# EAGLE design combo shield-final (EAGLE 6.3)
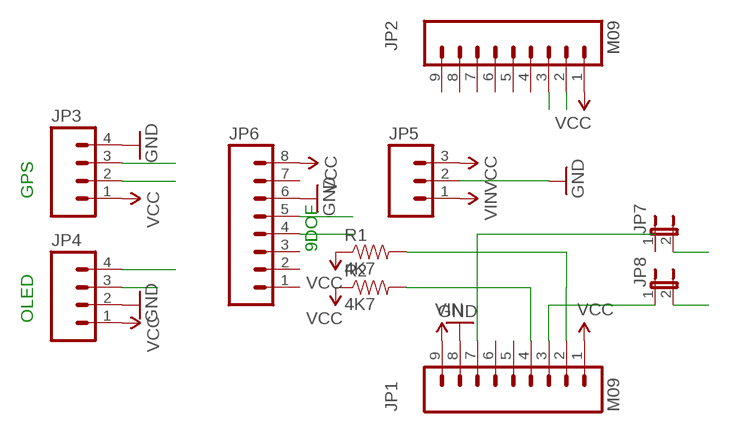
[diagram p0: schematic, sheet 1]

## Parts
JP1  M09  [1X09]
JP2  M09  [1X09]
JP3  M04PTH  [1X04]
JP4  M04PTH  [1X04]
JP5  M03PTH  [1X03]
JP6  M081X08  [1X08]
JP7  JUMPER-2SMD-NO  [SJ_2S-NO]
JP8  JUMPER-2SMD-NO  [SJ_2S-NO]
R1  4K7  RESISTORPTH-1/4W  [AXIAL-0.4]
R2  4K7  RESISTORPTH-1/4W  [AXIAL-0.4]

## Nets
GND [POWER]: JP1.8 JP3.4 JP4.2 JP5.2 JP6.6
N$2: JP1.3 JP8.1
N$3: JP1.7 JP7.1
RX: JP2.2 JP3.3 JP7.2
SCL: JP1.4 JP4.3 JP6.5 R2.P$2
SDA: JP1.2 JP4.4 JP6.4 R1.P$2
TX: JP2.3 JP3.2 JP8.2
VCC: JP1.1 JP2.1 JP3.1 JP4.1 JP5.3 JP6.8 R1.P$1 R2.P$1
VIN: JP1.9 JP5.1
Unconnected: JP1.5 JP1.6 JP2.4 JP2.5 JP2.6 JP2.7 JP2.8 JP2.9 JP6.1 JP6.2 JP6.3 JP6.7

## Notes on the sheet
- GPS
- 9DOF
- OLED

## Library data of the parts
JP1 JP2 = SparkFun:M09: Header 9 Standard 9-pin 0.1" header. Use with straight break away headers (SKU : PRT-00116), right angle break away headers (PRT-00553), swiss pins (PRT-00743), machine pins (PRT-00117), and female headers (PRT-00115).
JP3 JP4 = SparkFun-Connectors:M04: Header 4 Standard 4-pin 0.1" header. Use with straight break away headers (SKU : PRT-00116), right angle break away headers (PRT-00553), swiss pins (PRT-00743), machine pins (PRT-00117), and female headers (PRT-00115). Molex polarized connector foot print use with SKU : PRT-08231 with associated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
JP5 = SparkFun:M03: Header 3 Standard 3-pin 0.1" header. Use with straight break away headers (SKU : PRT-00116), right angle break away headers (PRT-00553), swiss pins (PRT-00743), machine pins (PRT-00117), and female headers (PRT-00115). Molex polarized connector foot print use with SKU : PRT-08232 with associated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
JP6 = SparkFun:M08: Header 8 Standard 8-pin 0.1" header. Use with straight break away headers (SKU : PRT-00116), right angle break away headers (PRT-00553), swiss pins (PRT-00743), machine pins (PRT-00117), and female headers (PRT-00115).
JP7 JP8 = SparkFun-Passives:JUMPER-2: Jumper
R1 R2 = SparkFun-Resistors:RESISTOR: Resistor

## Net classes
1 POWER: width 0.203 mm

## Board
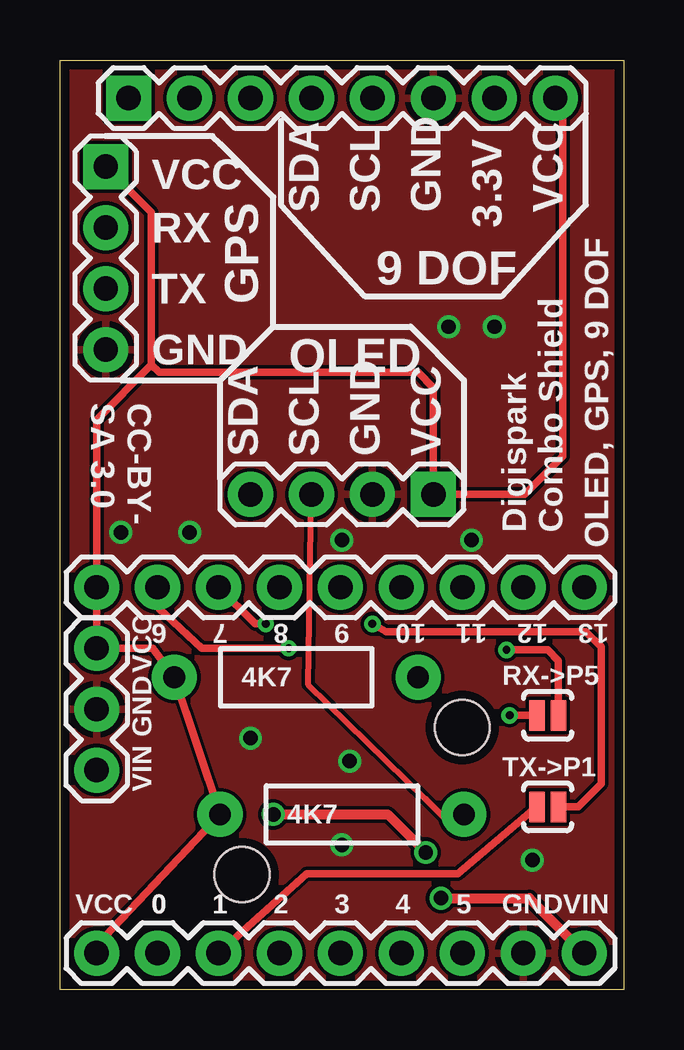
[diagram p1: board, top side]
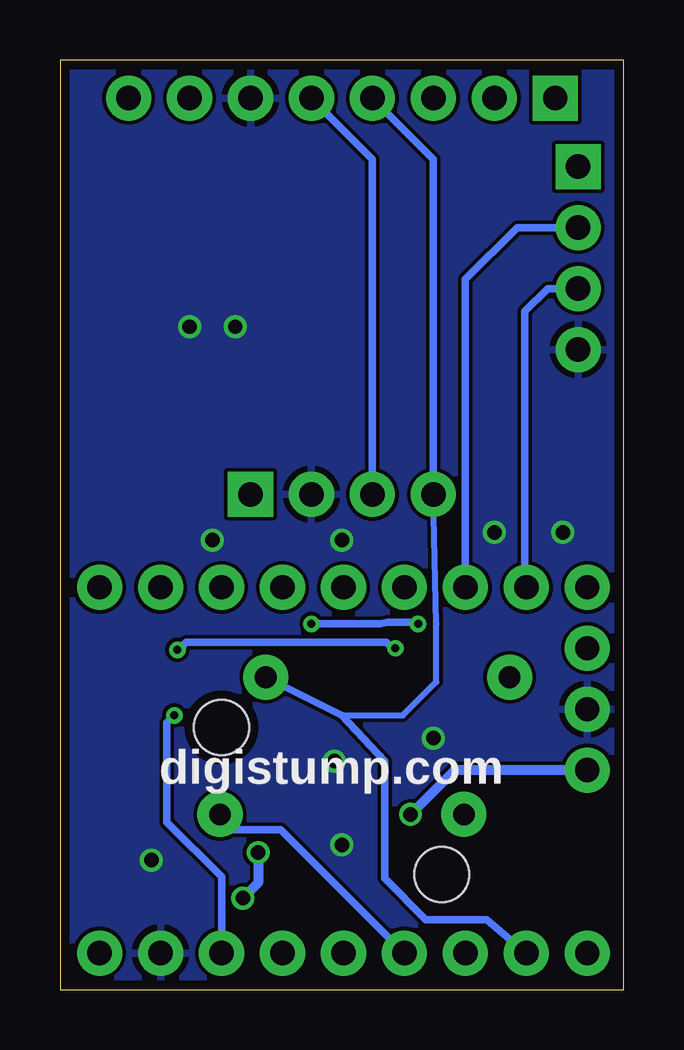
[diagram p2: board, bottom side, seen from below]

Size 23.5 x 38.73 mm. Coordinates in mm from the lower left corner, seen from the top.
Outline: 0,0 0,38.73 23.5,38.73 23.5,0 0,0
Copper layers (1*16): Top 0.0356mm / dielectric 1.5011mm / Bottom 0.0356mm
Design rules "eriks": minimum track width 6mil, minimum drill 13mil, track to track 6mil, track to pad 6mil, pad to pad 6mil, via to via 6mil, smd to smd 6mil, copper to edge 15mil, drill to drill 6mil, minimum pad ring 7mil, minimum via ring 7mil, stop-mask expansion 4mil, vias tented up to drill 20mil, thermal gap 10mil
Holes 2.29 mm at 16.76,10.92 7.59,4.79

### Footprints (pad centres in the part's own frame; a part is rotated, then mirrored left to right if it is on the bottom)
1X09 = drill 1.016 pad 1.88: 1 0,0; 2 2.54,0; 3 5.08,0; 4 7.62,0; 5 10.16,0; 6 12.7,0; 7 15.24,0; 8 17.78,0; 9 20.32,0
1X04 = drill 1.016 pad 1.88 square: 1 0,0 | drill 1.016 pad 1.88: 2 2.54,0; 3 5.08,0; 4 7.62,0
1X03 = drill 1.016 pad 1.88: 1 0,0; 2 2.54,0; 3 5.08,0
1X08 = drill 1.016 pad 1.88 square: 1 0,0 | drill 1.016 pad 1.88: 2 2.54,0; 3 5.08,0; 4 7.62,0; 5 10.16,0; 6 12.7,0; 7 15.24,0; 8 17.78,0
SJ_2S-NO = smd 0.635 x 1.27: 1 -0.45,0; 2 0.45,0
AXIAL-0.4 = drill 0.9 pad 1.88: P$1 -5.08,0; P$2 5.08,0

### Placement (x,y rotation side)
JP1  1.52,1.52 0 top
JP2  1.52,16.76 0 top
JP3  1.91,34.29 270 top
JP4  15.56,20.64 180 top
JP5  1.52,9.14 90 top
JP6  2.86,37.15 0 top
JP7  20.32,11.43 0 top
JP8  20.32,7.62 0 top
R1  9.84,13.02 0 top
R2  11.75,7.3 0 top

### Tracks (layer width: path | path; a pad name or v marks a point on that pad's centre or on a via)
GND  (via drill 0.6)
  other vias: 7.94,10.48 12.06,9.53 11.75,6.03 19.68,5.4 2.54,19.05 5.4,19.05 16.19,27.62 18.1,27.62 11.75,18.73 17.14,18.73
  pour Bottom: 0,38.73 0,0 23.5,0 23.5,38.73
  pour Top: 0,38.73 0,0 23.5,0 23.5,38.73
N$2
  Top 0.305: JP1.3 10.29,4.83 16.57,4.83 JP8.1
N$3  (via drill 0.33)
  Top 0.305: v18.73,11.43 JP7.1
  Bottom 0.305: JP1.7 16.76,4.7 19.05,6.99 19.05,11.11 v18.73,11.43
RX  (via drill 0.33)
  Top 0.305: JP7.2 20.77,13.71 20.32,14.16 v18.61,14.16 | v9.53,14.22 5.91,14.22 4.13,15.88 4.13,16.7 JP2.2
  Bottom 0.305: JP3.3 3.17,29.21 4.13,28.26 4.13,16.83 JP2.2 | v9.53,14.22 9.65,14.22 9.91,14.48 18.22,14.48 18.41,14.29 18.41,14.35 v18.61,14.16
SCL
  Top 0.254: R2.P$2 16.19,6.99 15.24,7.94 10.35,12.7 JP4.3
  Bottom 0.305: JP4.3 10.48,34.61 JP6.5 | JP1.4 14.29,6.67 16.51,6.67 R2.P$2
SDA
  Bottom 0.254: 11.75,11.43 9.21,11.43 7.81,12.83 7.81,15.24 JP4.4
  Bottom 0.305: JP4.4 7.94,34.61 JP6.4 | R1.P$2 11.75,11.43 9.97,9.53 9.97,4.64 8.26,2.92 5.71,2.92 JP1.2
TX  (via drill 0.33)
  Top 0.305: JP8.2 21.59,7.62 22.54,8.57 22.54,12.38 22.54,14.29 21.91,14.92 13.59,14.92 v13.02,15.24 | v8.57,15.24 8.13,15.24 JP2.3
  Bottom 0.305: JP2.3 6.6,29.59 4.45,31.75 JP3.2 | v13.02,15.24 10.16,15.24 9.84,15.3 8.89,15.3 v8.57,15.24
VCC
  Top 0.305: JP1.1 1.52,1.84 R2.P$1 R1.P$1 3.87,14.22 JP5.3 JP2.1 1.52,23.75 3.81,26.04 | 3.81,26.04 3.81,32.38 JP3.1 | JP6.8 20.95,36.83 20.95,22.23 19.37,20.64 JP4.1 15.56,25.08 14.92,25.72 4.13,25.72 3.81,26.04
VIN  (via drill 0.6)
  Top 0.406: v8.89,7.3 13.65,7.3 v15.24,5.71 | v15.88,3.81 19.56,3.81 JP1.9
  Bottom 0.406: JP5.1 7.05,9.14 v8.89,7.3 | v15.24,5.71 15.24,4.45 v15.88,3.81

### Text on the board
tPlace: VCC | SDA | SCL | GND | 3.3V | VCC | RX | 9 DOF | TX | GPS | GND | OLED | CC-BY- / SA 3.0 | SDA | SCL | GND | VCC | Digispark / Combo Shield | OLED, GPS, 9 DOF | 6 | 7 | 8 | 9 | 10 | 11 | 12 | 13 | VCC | RX->P5 | GND | TX->P1 | VIN | VCC | 0 | 0 | 1 | 2 | 3 | 4 | 5 | GND | VIN
bPlace: digistump.com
